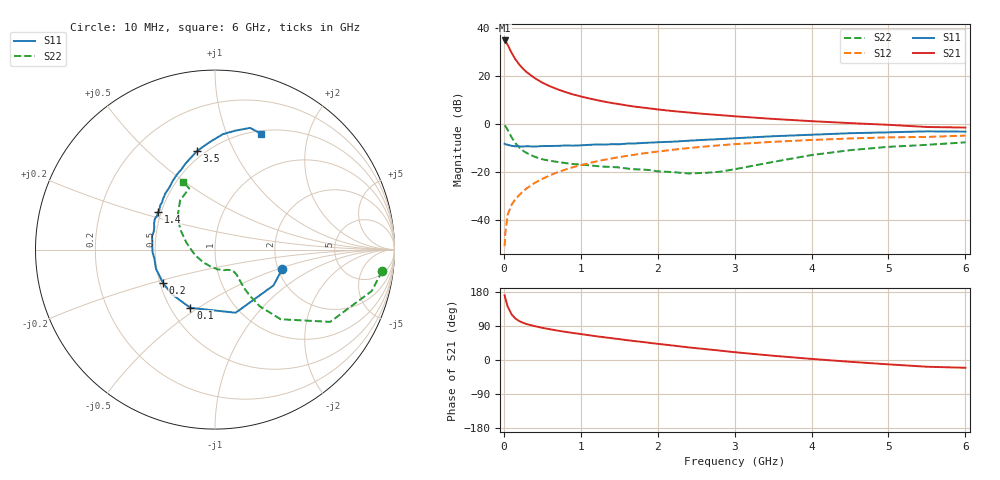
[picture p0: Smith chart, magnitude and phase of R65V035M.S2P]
! SIEMENS Small Signal Semiconductors
! BFR193
! Si NPN RF Bipolar Junction Transistor in SOT23
! VCE = 5 V  IC = 35 mA
! Common Emitter S-Parameters:  May  1996
# GHz  S  MA  R  50
!  f  S11  S21  S12  S22
! GHz  MAG  ANG  MAG  ANG  MAG  ANG  MAG  ANG
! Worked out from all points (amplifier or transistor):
!   36 points, 10 MHz to 6 GHz, reference 50 ohm
!   highest |S21| = 34.7 dB at 10 MHz (marker M1)
!   |S21| within 3 dB of that: start of sweep to 67.99 MHz
!   unconditionally stable (mu >= 1): 454.6 MHz to 2.011 GHz
!   at 250 MHz: K = 0.91, MSG = 25.4 dB, |S12| = -27.9 dB
!   at 1.4 GHz: K = 1.02, MAG = 10.6 dB, |S12| = -14.3 dB
!   at 6 GHz: K = 0.95, MSG = 1.7 dB, |S12| = -4.8 dB
!   S11 on the Smith chart (normalised r, x): 10 MHz: 2.10, -0.54; 100 MHz: 0.63, -0.46; 200 MHz: 0.52, -0.22; 1.4 GHz: 0.48, +0.24; 3.5 GHz: 0.46, +0.73; 6 GHz: 0.53, +1.33
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0.01  0.3896 -16.4  54.6 170.6  0.0029 85.5  0.9388 -7.3
0.02  0.3821 -31.5  52.66 162.1  0.0056 80.9  0.9033 -14.8
0.05  0.3701 -71.9  44.22 141.1  0.0131 69.9  0.7577 -32.1
0.1  0.3523 -112.9  30.44 120.7  0.021 66.7  0.5333 -46.7
0.15  0.3457 -133.5  22.18 109.4  0.0275 67.1  0.4027 -51.7
0.2  0.3445 -147.0  17.33 102.7  0.0333 69.1  0.3269 -52.9
0.25  0.3421 -155.6  14.05 98.2  0.0401 70.0  0.2784 -52.9
0.3  0.346 -161.8  11.87 94.6  0.0465 71.2  0.2488 -52.2
0.4  0.3415 -171.7  9.042 89.4  0.0596 72.3  0.2095 -50.7
0.5  0.3485 -177.9  7.258 84.9  0.0726 72.5  0.1852 -49.3
0.6  0.35 176.8  6.098 81.1  0.086 72.2  0.1723 -49.2
0.7  0.3523 172.3  5.267 77.5  0.0999 71.6  0.1632 -49.4
0.8  0.3586 168.1  4.623 74.3  0.1131 70.5  0.1547 -50.1
0.9  0.3558 163.3  4.131 71.2  0.1271 69.7  0.1477 -50.7
1.1  0.3691 157.0  3.436 65.6  0.1533 67.5  0.1395 -55.0
1.4  0.3813 146.3  2.74 57.6  0.1924 63.6  0.1286 -62.5
1.7  0.3952 138.2  2.307 49.9  0.2309 59.4  0.1146 -73.2
2.2  0.4302 126.1  1.859 38.1  0.293 52.2  0.1003 -100.5
3.5  0.5584 100.3  1.279 11.2  0.4273 32.1  0.1631 166.7
4.5  0.6452 86.0  1.047 -4.7  0.5022 18.0  0.2864 136.0
5.5  0.7057 73.9  0.869 -17.8  0.5402 4.1  0.3698 112.9
6  0.6951 68.5  0.846 -20.5  0.5757 0.1  0.4167 115.0
